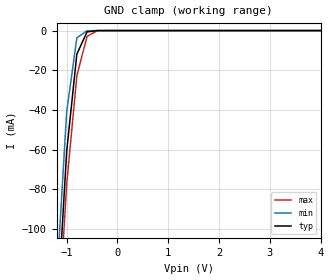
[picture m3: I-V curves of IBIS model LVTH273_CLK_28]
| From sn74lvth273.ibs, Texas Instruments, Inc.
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|   Model LVTH273_CLK_28
[Model]   LVTH273_CLK_28
Model_type  Input
Polarity   Non-Inverting
Vinl = 0.8
Vinh = 2.0
| variable   typ   min   max
C_comp   4pf   NA   NA
[Temperature Range]   40   -25   100
| Ambient temperatur   25   -40   85
[Voltage range]   2.8   2.7   2.9
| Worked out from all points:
|   GND clamp passes 1 mA (typ) near -0.61 V on its own axis
[GND Clamp]
|   Voltage   I(typ)   I(min)   I(max)
-5V       -2.439A    -2.779A    -2.169A
-1.2V     -148.5mA   -127.6mA   -163mA
-1V       -60.92mA   -40.94mA   -77.55mA
-800mV    -11.89mA   -3.666mA   -22.87mA
-600mV    -680.4uA   -95.57uA   -2.964mA
-400mV    -3.223uA   -117.9nA   -89.26uA
5V        327.8pA    281.4nA    297pA
